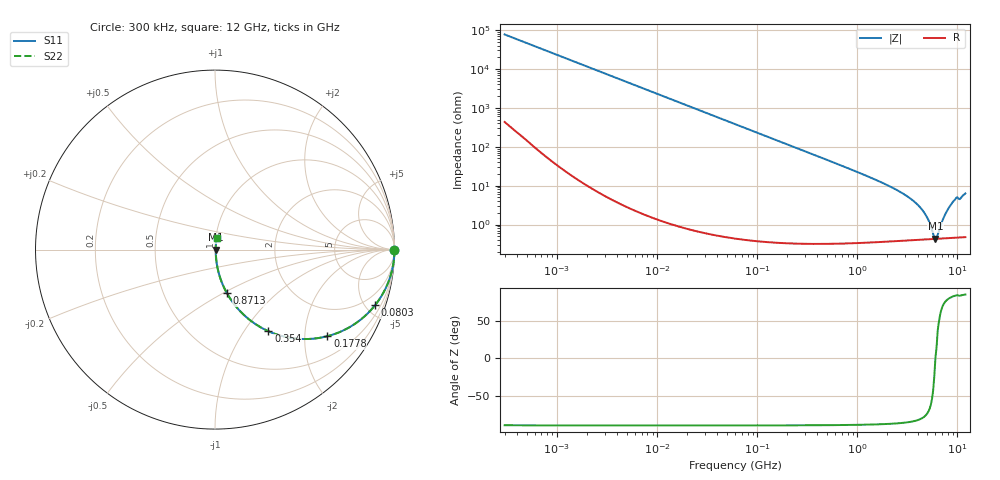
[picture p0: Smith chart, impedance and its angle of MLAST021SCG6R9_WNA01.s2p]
! MLAST021SCG6R9_WNA01  S-PARAMETER MODEL  ( General Type )
! Model Generated by TAIYO YUDEN Corporation (http://www.ty-top.com)
! Version 1.0
! TAIYO YUDEN Control No. 220901
! Copyright(c) 2022 TAIYO YUDEN CO.,LTD. All Rights Reserved.
! Product Description (link to TY-COMPAS)
! https://ds.yuden.co.jp/TYCOMPAS/or/detail?pn=MLAST021SCG6R9CWNA01&u=M
! Products Name : Multilayer Ceramic Capacitors
! Characteristics :
!  Capacitance : 6.9 pF , Rated Voltage : 25V , TCC : CG / C0G
!  Case Size : 0.25 x 0.125 / 0.0098 x 0.0049 [mm/inch] , Thickness : 0.125 / 0.0049 [mm/inch]
!  (Conditions: Temperature = 25 degC , DC Bias Current/Voltage = 0A / 0V)
! External Node Assignments :
!  1  o---| |---o  2
! GND o---------o GND
! Frequency Range : 0.3MHz  -  12000MHz  [ 401 STEP ]
# MHz S RI R 50
! Freq[MHz].  S11 Real  S11 Imag  S21 Real  S21 Imag  S12 Real  S12 Imag  S22 Real  S22 Imag
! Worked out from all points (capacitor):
!   401 points, 300 kHz to 12 GHz, reference 50 ohm
!   read as one part in series: C = 6.9 pF near 316.3 kHz
!   lowest |Z| = 431 mohm at 6.026 GHz (marker M1)
!   series resonance near 6.022 GHz, so ESL is about 100 pH
!   S11 on the Smith chart (normalised r, x): 300 kHz: open; 80.3 MHz: 1.01, -5.74; 177.8 MHz: 1.01, -2.59; 354 MHz: 1.01, -1.30; 871.3 MHz: 1.01, -0.52; 12 GHz: 1.01, +0.13
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0.3  1 -0.0013  9.03e-06 0.0013  9.03e-06 0.0013  1 -0.0013
1.769972  0.9999 -0.00767  6.6e-05 0.00767  6.6e-05 0.00767  0.9999 -0.00767
10.44266  0.9979 -0.0452  0.00207 0.0452  0.00207 0.0452  0.9979 -0.0452
27.10171  0.9863 -0.1159  0.0137 0.1159  0.0137 0.1159  0.9863 -0.1159
60  0.9364 -0.2435  0.0636 0.2435  0.0636 0.2435  0.9364 -0.2435
80.29859  0.8915 -0.3103  0.1085 0.3103  0.1085 0.3103  0.8915 -0.3103
177.7716  0.6266 -0.4824  0.3734 0.4824  0.3734 0.4824  0.6266 -0.4824
353.9943  0.2975 -0.4547  0.7025 0.4547  0.7025 0.4547  0.2975 -0.4547
540.8523  0.1537 -0.3569  0.8463 0.3569  0.8463 0.3569  0.1537 -0.3569
871.3074  0.0656 -0.2414  0.9344 0.2414  0.9344 0.2414  0.0656 -0.2414
2088.533  0.0129 -0.0955  0.9871 0.0955  0.9871 0.0955  0.0129 -0.0955
3107.553  0.0068 -0.0539  0.9932 0.0539  0.9932 0.0539  0.0068 -0.0539
4158.869  0.00489 -0.0287  0.9951 0.0287  0.9951 0.0287  0.00489 -0.0287
4875.354  0.00442 -0.0161  0.9956 0.0161  0.9956 0.0161  0.00442 -0.0161
5278.635  0.00431 -0.01  0.9957 0.01  0.9957 0.01  0.00431 -0.01
5715.274  0.00427 -0.00395  0.9957 0.00395  0.9957 0.00395  0.00427 -0.00395
6026.253  0.00429 5.55e-05  0.9957 -5.55e-05  0.9957 -5.55e-05  0.00429 5.55e-05
6354.153  0.00434 0.00337  0.9957 -0.00337  0.9957 -0.00337  0.00434 0.00337
7448.838  0.0047 0.0165  0.9953 -0.0165  0.9953 -0.0165  0.0047 0.0165
8732.115  0.00566 0.0336  0.9943 -0.0336  0.9943 -0.0336  0.00566 0.0336
9454.42  0.00645 0.0432  0.9935 -0.0432  0.9935 -0.0432  0.00645 0.0432
12000  0.00862 0.0621  0.9914 -0.0621  0.9914 -0.0621  0.00862 0.0621
